| IBIS file imx8qm_29x29_rev1_27_15charsmax.ibs
[IBIS Ver]   6.0
[Comment Char]   |_char
[File Name]   imx8qm_29x29_rev1_27_15charsmax.ibs
[File Rev]   1.27
[Date]   Mon Mar 15 02:13:26 2021
[Source]   NXP Viper 2020.06.15
[Notes]
[Disclaimer] IMPORTANT NOTICE
  This information is provided on an AS IS basis and without warranty.
  IN NO EVENT SHALL NXP BE LIABLE FOR INCIDENTAL OR CONSEQUENTIAL
  DAMAGES ARISING FROM USE OF THIS INFORMATION. THIS DISCLAIMER OF
  WARRANTY EXTENDS TO THE USER OF THE INFORMATION, AND TO THEIR CUSTOMERS
  OR USERS OF PRODUCTS  AND IS IN LIEU OF ALL WARRANTIES WHETHER EXPRESS,
  IMPLIED, OR STATUTORY, INCLUDING IMPLIED WARRANTIES OF MERCHANTABILITY
  OR FITNESS FOR PARTICULAR PURPOSE.
  NXP does not represent or warrant that the information furnished
  hereunder is free of infringement of any third party patents,
  copyrights, trade secrets, or other intellectual property rights.
  NXP does not represent or warrant that the information is free of
  defect, or that it meets any particular standard, requirements or need
  of the user of the infomation or their customers.
  NXP reserves the right to change the information in this file
  without notice.
   http://www.nxp.com
[Copyright]   (C) Copyright NXP 2004 - 2021, All Rights Reserved.
|   29x29
[Component]   29x29
[Manufacturer]   NXP
[Package]
| variable   typ   min   max
R_pkg   0.50181   0.071251   0.87203
L_pkg   3.032e-09   8.667e-10   5.190e-09
C_pkg   1.442e-12   7.770e-13   2.498e-12
[Pin] signal_name   model_name   R_pin   L_pin   C_pin
A3   VSS_MAIN   GND   NA   NA   NA
A5   USDHC1_RESET_B   BDPROGSCARUDQP_SDMMC_STD_3V3SF_FC_INNER  0.71494   4.208e-09 1.803e-12
A7   USDHC2_VSELECT   BDPROGSCARUDQP_SDMMC_STD_3V3SF_FC_OUTER  0.67873   4.010e-09 1.761e-12
A9   ENET0_MDC   BDPROGSCARUDQP_SDMMC_STD_3V3SF_FC_OUTER  0.67049   4.031e-09 1.735e-12
A11   ENET1_REFCLK_125M_25M   BDPROGSCARUDQP_SDMMC_STD_3V3SF_FC_OUTER  0.64637   3.820e-09 1.719e-12
A13   ENET1_MDC   BDPROGSCARUDQP_SDMMC_STD_3V3SF_FC_OUTER  0.66667   3.947e-09 1.724e-12
A15   PCIE_CTRL0_WAKE_B   BDPROGSCARUDQP_SDMMC_STD_3V3SF_FC_OUTER  0.65437   3.912e-09 1.725e-12
A17   PCIE_CTRL0_CLKREQ_B   BDPROGSCARUDQP_SDMMC_STD_3V3SF_FC_INNER  0.68404   4.044e-09 1.697e-12
A19   PCIE_SATA0_RX0_P   ABI_SERDES   0.65685   4.000e-09 1.482e-12
A21   PCIE1_RX0_P   ABI_SERDES   0.61374   3.771e-09 1.410e-12
A23   VSS_MAIN   GND   NA   NA   NA
A25   PCIE_CTRL1_CLKREQ_B   BDPROGSCARUDQP_SDMMC_STD_3V3SF_FC_OUTER  0.85097   5.022e-09 2.136e-12
A27   PCIE_CTRL1_WAKE_B   BDPROGSCARUDQP_SDMMC_STD_3V3SF_FC_INNER  0.87203   5.190e-09 2.111e-12
A29   PCIE0_RX0_P   ABI_SERDES   0.60799   3.796e-09 1.403e-12
A31   VSS_MAIN   GND   NA   NA   NA
A33   USB_SS3_TX_P   USB3_CDN   0.57069   3.681e-09 1.574e-12
A35   USB_OTG2_VBUS   NC   0.74136   4.399e-09 1.861e-12
A37   USB_OTG1_ID   NC   0.82585   4.889e-09 1.965e-12
A39   USB_OTG1_VBUS   hs_vbus_input   0.79385   4.631e-09 1.953e-12
A41   ENET0_RGMII_TXC   BDPROGSCARUDQP_SDMMC_STD_3V3SF_FC_INNER  0.63855   3.785e-09 1.694e-12
A43   ENET0_RGMII_TXD0   BDPROGSCARUDQP_SDMMC_STD_3V3SF_FC_INNER  0.63821   3.801e-09 1.640e-12
A45   ENET0_RGMII_TXD2   BDPROGSCARUDQP_SDMMC_STD_3V3SF_FC_INNER  0.68513   3.981e-09 1.746e-12
A47   ENET0_RGMII_RXD0   BDPROGSCARUDQP_SDMMC_STD_3V3SF_FC_INNER  0.70942   4.117e-09 1.762e-12
A49   ENET1_RGMII_TXD0   RGMII_TX   0.70216   4.118e-09 1.784e-12
A51   VSS_MAIN   GND   NA   NA   NA
B4   USDHC1_VSELECT   BDPROGSCARUDQP_SDMMC_STD_3V3SF_FC_OUTER  0.72105   4.248e-09 1.878e-12
B6   VSS_MAIN   GND   NA   NA   NA
B8   USDHC2_CD_B   BDPROGSCARUDQP_SDMMC_STD_3V3SF_FC_OUTER  0.65725   3.867e-09 1.789e-12
B10   ENET0_REFCLK_125M_25M   BDPROGSCARUDQP_SDMMC_STD_3V3SF_FC_INNER  0.62462   3.773e-09 1.701e-12
B12   VSS_MAIN   GND   NA   NA   NA
B14   VSS_MAIN   GND   NA   NA   NA
B16   PCIE_SATA0_TX0_P   ABI_SERDES   0.66405   4.087e-09 1.502e-12
B18   VSS_MAIN   GND   NA   NA   NA
B20   PCIE_SATA0_RX0_N   ABI_SERDES   0.65179   3.969e-09 1.493e-12
B22   PCIE1_RX0_N   ABI_SERDES   0.60933   3.642e-09 1.423e-12
B24   PCIE1_TX0_P   ABI_SERDES   0.54832   3.450e-09 1.344e-12
B26   PCIE0_TX0_P   ABI_SERDES   0.53719   3.375e-09 1.333e-12
B28   VSS_MAIN   GND   NA   NA   NA
B30   PCIE0_RX0_N   ABI_SERDES   0.60644   3.657e-09 1.420e-12
B32   USB_SS3_TX_N   USB3_CDN   0.56535   3.654e-09 1.559e-12
B34   USB_SS3_RX_N   USB3_CDN   0.57636   3.751e-09 1.628e-12
B36   VSS_MAIN   GND   NA   NA   NA
B38   USB_OTG2_DP   USB2_CDN   0.66542   4.197e-09 1.802e-12
B40   USB_OTG1_DP   USB2_NXP   0.68855   4.331e-09 1.847e-12
B42   ENET0_RGMII_TXD1   BDPROGSCARUDQP_SDMMC_STD_3V3SF_FC_OUTER  0.58126   3.465e-09 1.663e-12
B44   ENET0_RGMII_RXC   BDPROGSCARUDQP_SDMMC_STD_3V3SF_FC_INNER  0.59473   3.532e-09 1.657e-12
B46   VSS_MAIN   GND   NA   NA   NA
B48   ENET1_RGMII_TX_CTL   RGMII_TX   0.67806   3.966e-09 1.806e-12
B50   ENET1_RGMII_RXC   RGMII_RX   0.6658   3.913e-09 1.811e-12
C1   VSS_MAIN   GND   NA   NA   NA
C3   FLEXCAN2_RX   BDPROGSCARUDQP_SDMMC_STD_3V3SF_FC_INNER  0.73333   4.310e-09 1.872e-12
C5   FLEXCAN0_RX   BDPROGSCARUDQP_SDMMC_STD_3V3SF_FC_INNER  0.6572   3.880e-09 1.799e-12
C7   USDHC2_RESET_B   BDPROGSCARUDQP_SDMMC_STD_3V3SF_FC_INNER  0.64223   3.776e-09 1.718e-12
C9   VSS_MAIN   GND   NA   NA   NA
C11   VSS_MAIN   GND   NA   NA   NA
C13   ENET1_MDIO   BDPROGSCARUDQP_SDMMC_STD_3V3SF_FC_INNER  0.63159   3.805e-09 1.707e-12
C15   VSS_MAIN   GND   NA   NA   NA
C17   PCIE_SATA0_TX0_N   ABI_SERDES   0.66021   3.964e-09 1.538e-12
C19   VSS_MAIN   GND   NA   NA   NA
C21   VSS_MAIN   GND   NA   NA   NA
C23   VSS_MAIN   GND   NA   NA   NA
C25   PCIE1_TX0_N   ABI_SERDES   0.54592   3.335e-09 1.359e-12
C27   PCIE0_TX0_N   ABI_SERDES   0.53539   3.267e-09 1.337e-12
C29   VSS_MAIN   GND   NA   NA   NA
C31   VSS_MAIN   GND   NA   NA   NA
C33   VSS_MAIN   GND   NA   NA   NA
C35   USB_SS3_RX_P   USB3_CDN   0.578   3.655e-09 1.644e-12
C37   USB_OTG2_DN   USB2_CDN   0.65338   4.100e-09 1.813e-12
C39   USB_OTG1_DN   USB2_NXP   0.68253   4.301e-09 1.869e-12
C41   VSS_MAIN   GND   NA   NA   NA
C43   VSS_MAIN   GND   NA   NA   NA
C45   ENET0_RGMII_RXD2   BDPROGSCARUDQP_SDMMC_STD_3V3SF_FC_INNER  0.56865   3.382e-09 1.610e-12
C47   ENET1_RGMII_TXD1   RGMII_TX   0.58297   3.447e-09 1.661e-12
C49   VSS_MAIN   GND   NA   NA   NA
C51   ENET1_RGMII_RXD1   RGMII_RX   0.69982   4.106e-09 1.867e-12
C53   VSS_MAIN   GND   NA   NA   NA
D2   MLB_CLK   BDPROGSCARUDQP_SDMMC_STD_3V3SF_FC_INNER  0.71101   4.209e-09 1.875e-12
D6   VSS_MAIN   GND   NA   NA   NA
D8   USDHC2_WP   BDPROGSCARUDQP_SDMMC_STD_3V3SF_FC_INNER  0.62513   3.651e-09 1.684e-12
D10   ENET0_MDIO   BDPROGSCARUDQP_SDMMC_STD_3V3SF_FC_INNER  0.56625   3.378e-09 1.592e-12
D12   QSPI1A_DATA0   BDPROGSCARUDQP_SDMMC_STD_3V3SF_FC_OUTER  0.56144   3.424e-09 1.570e-12
D14   QSPI1A_DATA1   BDPROGSCARUDQP_SDMMC_STD_3V3SF_FC_INNER  0.53085   3.195e-09 1.560e-12
D16   VSS_MAIN   GND   NA   NA   NA
D18   VSS_MAIN   GND   NA   NA   NA
D20   PCIE_CTRL0_PERST_B   BDPROGSCARUDQP_SDMMC_STD_3V3SF_FC_INNER  0.51533   3.133e-09 1.473e-12
D22   PCIE_REXT   NC   0.50872   3.207e-09 1.487e-12
D24   VSS_MAIN   GND   NA   NA   NA
D26   VSS_MAIN   GND   NA   NA   NA
D28   VSS_MAIN   GND   NA   NA   NA
D30   MLB_SIG_P   mlb_data   0.47295   2.889e-09 1.375e-12
D32   MLB_CLK_P   mlb_clk   0.47306   2.904e-09 1.407e-12
D34   VSS_MAIN   GND   NA   NA   NA
D36   VSS_MAIN   GND   NA   NA   NA
D38   VSS_MAIN   GND   NA   NA   NA
D40   VSS_MAIN   GND   NA   NA   NA
D42   ENET0_RGMII_TXD3   BDPROGSCARUDQP_SDMMC_STD_3V3SF_FC_OUTER  0.54802   3.277e-09 1.536e-12
D44   ENET0_RGMII_RXD1   BDPROGSCARUDQP_SDMMC_STD_3V3SF_FC_OUTER  0.54964   3.286e-09 1.569e-12
D46   ENET1_RGMII_TXC   RGMII_TX   0.56118   3.341e-09 1.609e-12
D48   ENET1_RGMII_TXD3   RGMII_TX   0.5816   3.434e-09 1.601e-12
D52   ENET1_RGMII_RXD2   RGMII_RX   0.67008   3.934e-09 1.799e-12
E1   MLB_SIG   BDPROGSCARUDQP_SDMMC_STD_3V3SF_FC_INNER  0.70584   4.172e-09 1.785e-12
E3   MLB_DATA   BDPROGSCARUDQP_SDMMC_STD_3V3SF_FC_OUTER  0.63145   3.764e-09 1.730e-12
E5   FLEXCAN1_RX   BDPROGSCARUDQP_SDMMC_STD_3V3SF_FC_INNER  0.60931   3.644e-09 1.672e-12
E7   FLEXCAN2_TX   BDPROGSCARUDQP_SDMMC_STD_3V3SF_FC_OUTER  0.54072   3.256e-09 1.551e-12
E9   VSS_MAIN   GND   NA   NA   NA
E11   QSPI1A_DATA3   BDPROGSCARUDQP_SDMMC_STD_3V3SF_FC_INNER  0.55954   3.390e-09 1.553e-12
E13   QSPI1A_DATA2   BDPROGSCARUDQP_SDMMC_STD_3V3SF_FC_OUTER  0.4728   2.874e-09 1.442e-12
E15   QSPI0A_SS0_B   BDPROGSCARUDQP_SDMMC_STD_3V3SF_FC_OUTER  0.51682   3.144e-09 1.446e-12
E17   QSPI0A_SCLK   BDPROGSCARUDQP_SDMMC_STD_3V3SF_FC_OUTER  0.44693   2.747e-09 1.424e-12
E19   VSS_MAIN   GND   NA   NA   NA
E21   VSS_MAIN   GND   NA   NA   NA
E23   PCIE_REF_QR   NC   0.44778   2.848e-09 1.371e-12
E25   PCIE_SATA_REFCLK100M_N   NC   0.45847   2.806e-09 1.335e-12
E27   USB_SS3_REXT   NC   0.43403   2.914e-09 1.329e-12
E29   USB_OTG2_REXT   NC   0.3739   2.509e-09 1.226e-12
E31   MLB_SIG_N   mlb_data   0.47898   2.890e-09 1.386e-12
E33   MLB_CLK_N   mlb_clk   0.48026   2.897e-09 1.367e-12
E35   MLB_DATA_N   mlb_data   0.50267   3.023e-09 1.406e-12
E37   USDHC1_DATA0   BDPROGSCARUDQP_SDMMC_STD_3V3SF_FC_OUTER  0.45646   2.769e-09 1.352e-12
E39   USDHC1_DATA2   BDPROGSCARUDQP_SDMMC_STD_3V3SF_FC_OUTER  0.50466   3.021e-09 1.399e-12
E41   ENET0_RGMII_TX_CTL   BDPROGSCARUDQP_SDMMC_STD_3V3SF_FC_OUTER  0.57458   3.399e-09 1.597e-12
E43   ENET0_RGMII_RX_CTL   BDPROGSCARUDQP_SDMMC_STD_3V3SF_FC_OUTER  0.52405   3.152e-09 1.459e-12
E45   ENET0_RGMII_RXD3   BDPROGSCARUDQP_SDMMC_STD_3V3SF_FC_OUTER  0.51175   3.076e-09 1.491e-12
E47   VSS_MAIN   GND   NA   NA   NA
E49   ENET1_RGMII_RX_CTL   RGMII_RX   0.60279   3.566e-09 1.646e-12
E51   ENET1_RGMII_RXD0   RGMII_RX   0.65133   3.797e-09 1.745e-12
E53   ENET1_RGMII_RXD3   RGMII_RX   0.68907   3.974e-09 1.824e-12
F2   VSS_MAIN   GND   NA   NA   NA
F4   VSS_MAIN   GND   NA   NA   NA
F8   USB_SS3_TC2   BDPROGSCUDQP_EXT_FC_INNER   0.52001   3.184e-09 1.481e-12
F10   QSPI1A_SCLK   BDPROGSCARUDQP_SDMMC_STD_3V3SF_FC_INNER  0.55245   3.337e-09 1.549e-12
F12   VSS_MAIN   GND   NA   NA   NA
F14   QSPI0A_DATA1   BDPROGSCARUDQP_SDMMC_STD_3V3SF_FC_OUTER  0.45208   2.741e-09 1.409e-12
F16   QSPI0A_SS1_B   BDPROGSCARUDQP_SDMMC_STD_3V3SF_FC_INNER  0.48133   2.964e-09 1.408e-12
F18   QSPI0B_SCLK   BDPROGSCARUDQP_SDMMC_STD_3V3SF_FC_INNER  0.39244   2.436e-09 1.330e-12
F20   QSPI0B_DATA3   BDPROGSCARUDQP_SDMMC_STD_3V3SF_FC_INNER  0.4028   2.469e-09 1.293e-12
F22   QSPI0B_SS0_B   BDPROGSCARUDQP_SDMMC_STD_3V3SF_FC_INNER  0.39427   2.450e-09 1.281e-12
F24   VSS_MAIN   GND   NA   NA   NA
F26   PCIE_SATA_REFCLK100M_P   NC   0.45666   2.807e-09 1.394e-12
F28   USB_HSIC0_STROBE   hsic   0.39203   2.462e-09 1.309e-12
F30   USB_OTG2_ID   NC   0.34712   2.212e-09 1.234e-12
F32   VSS_MAIN   GND   NA   NA   NA
F34   MLB_DATA_P   mlb_data   0.49658   3.005e-09 1.415e-12
F36   VSS_MAIN   GND   NA   NA   NA
F38   USDHC1_DATA1   BDPROGSCARUDQP_SDMMC_STD_3V3SF_FC_INNER  0.46305   2.802e-09 1.318e-12
F40   USDHC1_DATA3   BDPROGSCARUDQP_SDMMC_STD_3V3SF_FC_INNER  0.50226   3.028e-09 1.440e-12
F42   USDHC1_DATA6   BDPROGSCARUDQP_SDMMC_STD_3V3SF_FC_OUTER  0.47942   2.912e-09 1.417e-12
F44   VSS_MAIN   GND   NA   NA   NA
F46   USDHC2_CLK   BDPROGSCARUDQP_SDMMC_STD_3V3SF_FC_INNER  0.67177   4.003e-09 1.796e-12
F50   VSS_MAIN   GND   NA   NA   NA
F52   VSS_MAIN   GND   NA   NA   NA
G1   DDR_CH1_DQ05   PDDRIO_PAD_DATA   0.66326   3.933e-09 1.688e-12
G3   DDR_CH1_DQ06   PDDRIO_PAD_DATA   0.63448   3.859e-09 1.718e-12
G5   VSS_MAIN   GND   NA   NA   NA
G7   FLEXCAN1_TX   BDPROGSCARUDQP_SDMMC_STD_3V3SF_FC_OUTER  0.54812   3.301e-09 1.588e-12
G9   VSS_MAIN   GND   NA   NA   NA
G11   QSPI1A_SS1_B   BDPROGSCARUDQP_SDMMC_STD_3V3SF_FC_OUTER  0.48621   2.959e-09 1.523e-12
G13   QSPI0A_DATA0   BDPROGSCARUDQP_SDMMC_STD_3V3SF_FC_INNER  0.46056   2.802e-09 1.455e-12
G15   VSS_MAIN   GND   NA   NA   NA
G17   QSPI0A_DQS   BDPROGSCARUDQP_SDMMC_STD_3V3SF_FC_INNER  0.37077   2.353e-09 1.286e-12
G19   QSPI0B_DATA2   BDPROGSCARUDQP_SDMMC_STD_3V3SF_FC_OUTER  0.3765   2.329e-09 1.271e-12
G21   VSS_MAIN   GND   NA   NA   NA
G23   VSS_MAIN   GND   NA   NA   NA
G25   PCIE_CTRL1_PERST_B   BDPROGSCARUDQP_SDMMC_STD_3V3SF_FC_OUTER  0.33043   2.156e-09 1.186e-12
G27   VSS_MAIN   GND   NA   NA   NA
G29   EMMC0_DATA0   BDPROGSCARUDQP_SDMMC_STD_3V3SF_FC_INNER  0.412   2.597e-09 1.278e-12
G31   EMMC0_DATA2   BDPROGSCARUDQP_SDMMC_STD_3V3SF_FC_INNER  0.37909   2.358e-09 1.243e-12
G33   VSS_MAIN   GND   NA   NA   NA
G35   EMMC0_DATA7   BDPROGSCARUDQP_SDMMC_STD_3V3SF_FC_OUTER  0.35183   2.211e-09 1.183e-12
G37   EMMC0_STROBE   BDPROGSCARUDQP_SDMMC_STD_3V3SF_FC_INNER  0.37074   2.314e-09 1.244e-12
G39   VSS_MAIN   GND   NA   NA   NA
G41   USDHC1_CMD   BDPROGSCARUDQP_SDMMC_STD_3V3SF_FC_INNER  0.49738   2.969e-09 1.475e-12
G43   USDHC1_DATA5   BDPROGSCARUDQP_SDMMC_STD_3V3SF_FC_INNER  0.51832   3.079e-09 1.500e-12
G45   USDHC2_DATA1   BDPROGSCARUDQP_SDMMC_STD_3V3SF_FC_OUTER  0.5606   3.400e-09 1.610e-12
G47   ENET1_RGMII_TXD2   RGMII_TX   0.55697   3.297e-09 1.553e-12
G49   VSS_MAIN   GND   NA   NA   NA
G51   DDR_CH0_DQ06   PDDRIO_PAD_DATA   0.63199   3.750e-09 1.739e-12
G53   DDR_CH0_DQ05   PDDRIO_PAD_DATA   0.66027   3.881e-09 1.779e-12
H2   DDR_CH1_DM0   PDDRIO_PAD_DATA   0.62675   3.725e-09 1.662e-12
H4   DDR_CH1_DQ04   PDDRIO_PAD_DATA   0.56957   3.379e-09 1.592e-12
H6   FLEXCAN0_TX   BDPROGSCARUDQP_SDMMC_STD_3V3SF_FC_OUTER  0.53476   3.306e-09 1.585e-12
H10   USB_SS3_TC3   BDPROGSCUDQP_EXT_FC_OUTER   0.43538   2.704e-09 1.347e-12
H12   QSPI1A_DQS   BDPROGSCARUDQP_SDMMC_STD_3V3SF_FC_OUTER  0.43856   2.706e-09 1.408e-12
H14   QSPI0A_DATA2   BDPROGSCARUDQP_SDMMC_STD_3V3SF_FC_INNER  0.42256   2.614e-09 1.399e-12
H16   QSPI0A_DATA3   BDPROGSCARUDQP_SDMMC_STD_3V3SF_FC_OUTER  0.40728   2.516e-09 1.306e-12
H18   QSPI0B_DATA0   BDPROGSCARUDQP_SDMMC_STD_3V3SF_FC_OUTER  0.34663   2.215e-09 1.213e-12
H20   QSPI0B_DATA1   BDPROGSCARUDQP_SDMMC_STD_3V3SF_FC_INNER  0.31327   1.955e-09 1.168e-12
H22   QSPI0B_DQS   BDPROGSCARUDQP_SDMMC_STD_3V3SF_FC_OUTER  0.306   1.964e-09 1.132e-12
H24   QSPI0B_SS1_B   BDPROGSCARUDQP_SDMMC_STD_3V3SF_FC_OUTER  0.34933   2.209e-09 1.161e-12
H26   USB_HSIC0_DATA   hsic   0.29076   1.955e-09 1.108e-12
H28   EMMC0_CLK   BDPROGSCARUDQP_SDMMC_STD_3V3SF_FC_INNER  0.40001   2.468e-09 1.271e-12
H30   EMMC0_DATA1   BDPROGSCARUDQP_SDMMC_STD_3V3SF_FC_OUTER  0.35924   2.228e-09 1.208e-12
H32   EMMC0_DATA3   BDPROGSCARUDQP_SDMMC_STD_3V3SF_FC_OUTER  0.30585   1.968e-09 1.176e-12
H34   EMMC0_DATA5   BDPROGSCARUDQP_SDMMC_STD_3V3SF_FC_OUTER  0.33315   2.092e-09 1.130e-12
H36   EMMC0_DATA6   BDPROGSCARUDQP_SDMMC_STD_3V3SF_FC_INNER  0.35261   2.188e-09 1.178e-12
H38   EMMC0_RESET_B   BDPROGSCARUDQP_SDMMC_STD_3V3SF_FC_OUTER  0.38186   2.351e-09 1.248e-12
H40   USDHC1_DATA4   BDPROGSCARUDQP_SDMMC_STD_3V3SF_FC_OUTER  0.4384   2.664e-09 1.395e-12
H42   USDHC1_DATA7   BDPROGSCARUDQP_SDMMC_STD_3V3SF_FC_INNER  0.44709   2.716e-09 1.362e-12
H44   USDHC2_CMD   BDPROGSCARUDQP_SDMMC_STD_3V3SF_FC_OUTER  0.54162   3.262e-09 1.572e-12
H48   USDHC2_DATA0   BDPROGSCARUDQP_SDMMC_STD_3V3SF_FC_INNER  0.62353   3.680e-09 1.694e-12
H50   DDR_CH0_DQ04   PDDRIO_PAD_DATA   0.56734   3.363e-09 1.592e-12
H52   DDR_CH0_DM0   PDDRIO_PAD_DATA   0.62698   3.731e-09 1.687e-12
J1   VSS_MAIN   GND   NA   NA   NA
J3   VSS_MAIN   GND   NA   NA   NA
J5   VSS_MAIN   GND   NA   NA   NA
J7   VSS_MAIN   GND   NA   NA   NA
J9   USB_SS3_TC0   BDPROGSCUDQP_EXT_FC_INNER   0.42059   2.620e-09 1.335e-12
J11   QSPI1A_SS0_B   BDPROGSCARUDQP_SDMMC_STD_3V3SF_FC_INNER  0.49996   3.013e-09 1.556e-12
J13   VSS_MAIN   GND   NA   NA   NA
J15   VSS_MAIN   GND   NA   NA   NA
J17   VSS_MAIN   GND   NA   NA   NA
J19   VSS_MAIN   GND   NA   NA   NA
J21   VSS_MAIN   GND   NA   NA   NA
J23   VSS_MAIN   GND   NA   NA   NA
J25   VSS_MAIN   GND   NA   NA   NA
J27   EMMC0_CMD   BDPROGSCARUDQP_SDMMC_STD_3V3SF_FC_OUTER  0.37925   2.371e-09 1.227e-12
J29   VSS_MAIN   GND   NA   NA   NA
J31   VSS_MAIN   GND   NA   NA   NA
J33   EMMC0_DATA4   BDPROGSCARUDQP_SDMMC_STD_3V3SF_FC_INNER  0.31324   1.999e-09 1.165e-12
J35   VSS_MAIN   GND   NA   NA   NA
J37   VSS_MAIN   GND   NA   NA   NA
J39   USDHC1_CLK   BDPROGSCARUDQP_SDMMC_STD_3V3SF_FC_OUTER  0.38556   2.407e-09 1.236e-12
J41   VSS_MAIN   GND   NA   NA   NA
J43   USDHC1_STROBE   BDPROGSCARUDQP_SDMMC_STD_3V3SF_FC_OUTER  0.49046   2.949e-09 1.423e-12
J45   USDHC2_DATA3   BDPROGSCARUDQP_SDMMC_STD_3V3SF_FC_OUTER  0.52798   3.184e-09 1.404e-12
J47   VSS_MAIN   GND   NA   NA   NA
J49   VSS_MAIN   GND   NA   NA   NA
J51   VSS_MAIN   GND   NA   NA   NA
J53   VSS_MAIN   GND   NA   NA   NA
K2   DDR_CH1_DQS0_P   PDQS_PAD   0.72024   4.233e-09 1.841e-12
K4   DDR_CH1_DQ09   PDDRIO_PAD_DATA   0.54194   3.298e-09 1.528e-12
K6   DDR_CH1_DQ03   PDDRIO_PAD_DATA   0.48681   2.954e-09 1.443e-12
K8   VSS_MAIN   GND   NA   NA   NA
K12   VSS_MAIN   GND   NA   NA   NA
K14   VSS_MAIN   GND   NA   NA   NA
K16   VSS_MAIN   GND   NA   NA   NA
K18   VSS_MAIN   GND   NA   NA   NA
K20   VSS_MAIN   GND   NA   NA   NA
K22   VSS_MAIN   GND   NA   NA   NA
K24   VSS_MAIN   GND   NA   NA   NA
K26   VSS_MAIN   GND   NA   NA   NA
K28   VSS_MAIN   GND   NA   NA   NA
K30   VSS_MAIN   GND   NA   NA   NA
K32   VSS_MAIN   GND   NA   NA   NA
K34   VSS_MAIN   GND   NA   NA   NA
K36   VSS_MAIN   GND   NA   NA   NA
K38   VSS_MAIN   GND   NA   NA   NA
K40   VSS_MAIN   GND   NA   NA   NA
K42   VSS_MAIN   GND   NA   NA   NA
K46   VSS_MAIN   GND   NA   NA   NA
K48   DDR_CH0_DQ03   PDDRIO_PAD_DATA   0.48777   2.944e-09 1.414e-12
K50   DDR_CH0_DQ09   PDDRIO_PAD_DATA   0.54335   3.312e-09 1.488e-12
K52   DDR_CH0_DQS0_P   PDQS_PAD   0.72197   4.255e-09 1.844e-12
L1   DDR_CH1_DQS0_N   PDQS_PAD   0.72434   4.328e-09 1.757e-12
L3   DDR_CH1_DQ11   PDDRIO_PAD_DATA   0.59817   3.687e-09 1.610e-12
L5   DDR_CH1_DQ08   PDDRIO_PAD_DATA   0.48028   2.943e-09 1.425e-12
L7   DDR_CH1_DQ02   PDDRIO_PAD_DATA   0.45079   2.788e-09 1.323e-12
L9   USB_SS3_TC1   BDPROGSCUDQP_EXT_FC_OUTER   0.39437   2.514e-09 1.317e-12
L11   VSS_MAIN   GND   NA   NA   NA
L13   VSS_MAIN   GND   NA   NA   NA
L15   VSS_MAIN   GND   NA   NA   NA
L17   VSS_MAIN   GND   NA   NA   NA
L19   VSS_MAIN   GND   NA   NA   NA
L21   VSS_MAIN   GND   NA   NA   NA
L23   VSS_MAIN   GND   NA   NA   NA
L25   VSS_MAIN   GND   NA   NA   NA
L27   VSS_MAIN   GND   NA   NA   NA
L29   VSS_MAIN   GND   NA   NA   NA
L31   VSS_MAIN   GND   NA   NA   NA
L33   VSS_MAIN   GND   NA   NA   NA
L35   VSS_MAIN   GND   NA   NA   NA
L37   VSS_MAIN   GND   NA   NA   NA
L39   VSS_MAIN   GND   NA   NA   NA
L41   VSS_MAIN   GND   NA   NA   NA
L43   VSS_MAIN   GND   NA   NA   NA
L45   USDHC2_DATA2   BDPROGSCARUDQP_SDMMC_STD_3V3SF_FC_INNER  0.45871   2.725e-09 1.411e-12
L47   DDR_CH0_DQ02   PDDRIO_PAD_DATA   0.45083   2.841e-09 1.355e-12
L49   DDR_CH0_DQ08   PDDRIO_PAD_DATA   0.48155   2.926e-09 1.418e-12
L51   DDR_CH0_DQ11   PDDRIO_PAD_DATA   0.59934   3.648e-09 1.622e-12
L53   DDR_CH0_DQS0_N   PDQS_PAD   0.7235   4.319e-09 1.771e-12
M2   VSS_MAIN   GND   NA   NA   NA
M4   VSS_MAIN   GND   NA   NA   NA
M6   VSS_MAIN   GND   NA   NA   NA
M8   VSS_MAIN   GND   NA   NA   NA
M10   VSS_MAIN   GND   NA   NA   NA
M14   VDD_MLB_DIG_1P8_3P3   POWER   NA   NA   NA
M16   VDD_USB_SS3_TC_3P3   POWER   NA   NA   NA
M18   VDD_QSPI1A_1P8_3P3   POWER   NA   NA   NA
M20   PCIE_SATA0_PHY_PLL_REF_RETURN   GND   0.078076  8.883e-10 2.121e-12
M22   VDD_PCIE1_PLL_1P8   POWER   NA   NA   NA
M24   VDD_PCIE_SATA0_1P0   POWER   NA   NA   NA
M26   VDD_PCIE0_1P0   POWER   NA   NA   NA
M28   PCIE0_PHY_PLL_REF_RETURN   GND   0.090376  9.966e-10 1.927e-12
M30   VDD_USB_SS3_LDO_1P0_CAP   POWER   NA   NA   NA
M32   VDD_USB_OTG1_1P0   POWER   NA   NA   NA
M34   VDD_USB_OTG2_3P3   POWER   NA   NA   NA
M36   VDD_USDHC1_1P8_3P3   POWER   NA   NA   NA
M38   VDD_USDHC2_1P8_3P3   POWER   NA   NA   NA
M40   VDD_ENET0_1P8_2P5_3P3   POWER   NA   NA   NA
M44   VSS_MAIN   GND   NA   NA   NA
M46   VSS_MAIN   GND   NA   NA   NA
M48   VSS_MAIN   GND   NA   NA   NA
M50   VSS_MAIN   GND   NA   NA   NA
M52   VSS_MAIN   GND   NA   NA   NA
N1   DDR_CH1_DQS1_P   PDQS_PAD   0.6386   3.872e-09 1.642e-12
N3   DDR_CH1_DQ10   PDDRIO_PAD_DATA   0.54172   3.267e-09 1.538e-12
N5   DDR_CH1_DQ13   PDDRIO_PAD_DATA   0.45905   2.855e-09 1.364e-12
N7   DDR_CH1_DM1   PDDRIO_PAD_DATA   0.3749   2.404e-09 1.248e-12
N9   DDR_CH1_DQ01   PDDRIO_PAD_DATA   0.31995   2.039e-09 1.116e-12
N11   DDR_CH1_DQ07   PDDRIO_PAD_DATA   0.23187   1.570e-09 9.871e-13
N13   VSS_MAIN   GND   NA   NA   NA
N15   VDD_FLEXCAN_1P8_3P3   POWER   NA   NA   NA
N17   VDD_ENET_MDIO_1P8_2P5_3P3   POWER   NA   NA   NA
N19   VDD_QSPI0_1P8_3P3   POWER   NA   NA   NA
N21   VDD_PCIE_SATA0_PLL_1P8   POWER   NA   NA   NA
N23   PCIE1_PHY_PLL_REF_RETURN   GND   0.072195  9.525e-10 1.343e-12
N25   VDD_PCIE1_1P0   POWER   NA   NA   NA
N27   VDD_PCIE0_PLL_1P8   POWER   NA   NA   NA
N29   VDD_PCIE_LDO_1P0_CAP   POWER   NA   NA   NA
N31   VDD_USB_OTG2_1P0   POWER   NA   NA   NA
N33   VDD_USB_OTG1_3P3   POWER   NA   NA   NA
N35   VDD_EMMC0_1P8_3P3   POWER   NA   NA   NA
N37   VDD_USDHC1_1P8_3P3   POWER   NA   NA   NA
N39   VDD_ENET0_1P8_2P5_3P3   POWER   NA   NA   NA
N41   VSS_MAIN   GND   NA   NA   NA
N43   DDR_CH0_DQ07   PDDRIO_PAD_DATA   0.22999   1.544e-09 9.890e-13
N45   DDR_CH0_DQ01   PDDRIO_PAD_DATA   0.32072   2.032e-09 1.120e-12
N47   DDR_CH0_DM1   PDDRIO_PAD_DATA   0.37407   2.370e-09 1.247e-12
N49   DDR_CH0_DQ13   PDDRIO_PAD_DATA   0.46598   2.903e-09 1.391e-12
N51   DDR_CH0_DQ10   PDDRIO_PAD_DATA   0.54312   3.246e-09 1.498e-12
N53   DDR_CH0_DQS1_P   PDQS_PAD   0.63588   3.825e-09 1.623e-12
P2   DDR_CH1_DQS1_N   PDQS_PAD   0.62973   3.778e-09 1.665e-12
P4   DDR_CH1_DQ14   PDDRIO_PAD_DATA   0.47322   2.923e-09 1.416e-12
P6   DDR_CH1_DQ15   PDDRIO_PAD_DATA   0.41122   2.633e-09 1.290e-12
P8   DDR_CH1_DQ12   PDDRIO_PAD_DATA   0.31879   2.070e-09 1.140e-12
P10   DDR_CH1_DQ00   PDDRIO_PAD_DATA   0.26612   1.777e-09 1.004e-12
P12   VSS_MAIN   GND   NA   NA   NA
P42   VSS_MAIN   GND   NA   NA   NA
P44   DDR_CH0_DQ00   PDDRIO_PAD_DATA   0.26606   1.803e-09 9.926e-13
P46   DDR_CH0_DQ12   PDDRIO_PAD_DATA   0.31564   1.974e-09 1.142e-12
P48   DDR_CH0_DQ15   PDDRIO_PAD_DATA   0.42142   2.670e-09 1.295e-12
P50   DDR_CH0_DQ14   PDDRIO_PAD_DATA   0.47632   2.946e-09 1.401e-12
P52   DDR_CH0_DQS1_N   PDQS_PAD   0.6299   3.763e-09 1.657e-12
R1   VSS_MAIN   GND   NA   NA   NA
R3   VSS_MAIN   GND   NA   NA   NA
R5   VSS_MAIN   GND   NA   NA   NA
R7   VSS_MAIN   GND   NA   NA   NA
R9   VSS_MAIN   GND   NA   NA   NA
R11   VSS_MAIN   GND   NA   NA   NA
R15   VSS_MAIN   GND   NA   NA   NA
R17   VSS_MAIN   GND   NA   NA   NA
R19   VSS_MAIN   GND   NA   NA   NA
R21   VSS_MAIN   GND   NA   NA   NA
R23   VSS_MAIN   GND   NA   NA   NA
R25   VSS_MAIN   GND   NA   NA   NA
R27   VSS_MAIN   GND   NA   NA   NA
R29   VSS_MAIN   GND   NA   NA   NA
R31   VSS_MAIN   GND   NA   NA   NA
R33   VSS_MAIN   GND   NA   NA   NA
R35   VSS_MAIN   GND   NA   NA   NA
R37   VSS_MAIN   GND   NA   NA   NA
R39   VSS_MAIN   GND   NA   NA   NA
R43   VSS_MAIN   GND   NA   NA   NA
R45   VSS_MAIN   GND   NA   NA   NA
R47   VSS_MAIN   GND   NA   NA   NA
R49   VSS_MAIN   GND   NA   NA   NA
R51   VSS_MAIN   GND   NA   NA   NA
R53   VSS_MAIN   GND   NA   NA   NA
T2   DDR_CH1_DCF09   PDDRIO_PAD_COMMAND   0.54813   3.276e-09 1.456e-12
T4   DDR_CH1_DCF10   PDDRIO_PAD_COMMAND   0.45838   2.772e-09 1.396e-12
T6   DDR_CH1_DCF08   PDDRIO_PAD_COMMAND   0.4138   2.542e-09 1.341e-12
T8   DDR_CH1_DCF13   PDDRIO_PAD_COMMAND   0.37803   2.393e-09 1.184e-12
T10   DDR_CH1_DTO1   PDDRIO_PAD_COMMAND   0.32279   2.073e-09 1.114e-12
T12   VSS_MAIN   GND   NA   NA   NA
T16   VSS_MAIN   GND   NA   NA   NA
T18   VDD_USDHC_VSELECT_1P8_3P3   POWER   NA   NA   NA
T20   VSS_MAIN   GND   NA   NA   NA
T22   VDD_PCIE_DIG_1P8_3P3   POWER   NA   NA   NA
T24   VSS_MAIN   GND   NA   NA   NA
T26   VDD_PCIE_IOB_1P8   POWER   NA   NA   NA
T28   VSS_MAIN   GND   NA   NA   NA
T30   VDD_MLB_1P8   POWER   NA   NA   NA
T32   VSS_MAIN   GND   NA   NA   NA
T34   VDD_MAIN   POWER   NA   NA   NA
T36   VSS_MAIN   GND   NA   NA   NA
T38   VDD_ENET1_1P8_2P5_3P3   POWER   NA   NA   NA
T42   VSS_MAIN   GND   NA   NA   NA
T44   DDR_CH0_DTO1   PDDRIO_PAD_COMMAND   0.32378   2.069e-09 1.115e-12
T46   DDR_CH0_DCF13   PDDRIO_PAD_COMMAND   0.37542   2.342e-09 1.191e-12
T48   DDR_CH0_DCF08   PDDRIO_PAD_COMMAND   0.41391   2.551e-09 1.300e-12
T50   DDR_CH0_DCF10   PDDRIO_PAD_COMMAND   0.45654   2.774e-09 1.396e-12
T52   DDR_CH0_DCF09   PDDRIO_PAD_COMMAND   0.54626   3.230e-09 1.570e-12
U1   DDR_CH1_DCF16   PDDRIO_PAD_COMMAND   0.54739   3.303e-09 1.529e-12
U3   DDR_CH1_DCF11   PDDRIO_PAD_COMMAND   0.5197   3.133e-09 1.489e-12
U5   DDR_CH1_DCF12   PDDRIO_PAD_COMMAND   0.42237   2.576e-09 1.387e-12
U7   DDR_CH1_DCF00   PDDRIO_PAD_COMMAND   0.35953   2.250e-09 1.250e-12
U9   DDR_CH1_DTO0   PDDRIO_PAD_COMMAND   0.24832   1.674e-09 9.811e-13
U11   DDR_CH1_VREF   NC   0.071251  8.720e-10 2.474e-12
U15   VDD_DDR_CH1_VDDQ   POWER   NA   NA   NA
U17   VSS_MAIN   GND   NA   NA   NA
U19   VDD_MAIN   POWER   NA   NA   NA
U21   VSS_MAIN   GND   NA   NA   NA
U23   VDD_MAIN   POWER   NA   NA   NA
U25   VDD_ANA1_1P8   POWER   NA   NA   NA
U27   VDD_PCIE_LDO_1P8   POWER   NA   NA   NA
U29   VDD_ANA0_1P8   POWER   NA   NA   NA
U31   VDD_ANA0_1P8   POWER   NA   NA   NA
U33   VSS_MAIN   GND   NA   NA   NA
U35   VDD_GPU1   POWER   NA   NA   NA
U37   VSS_MAIN   GND   NA   NA   NA
U39   VDD_DDR_CH0_VDDQ   POWER   NA   NA   NA
U43   DDR_CH0_VREF   NC   0.072272  8.667e-10 2.439e-12
U45   DDR_CH0_DTO0   PDDRIO_PAD_COMMAND   0.24706   1.642e-09 9.813e-13
U47   DDR_CH0_DCF00   PDDRIO_PAD_COMMAND   0.35996   2.249e-09 1.228e-12
U49   DDR_CH0_DCF12   PDDRIO_PAD_COMMAND   0.42158   2.584e-09 1.355e-12
U51   DDR_CH0_DCF11   PDDRIO_PAD_COMMAND   0.51885   3.098e-09 1.498e-12
U53   DDR_CH0_DCF16   PDDRIO_PAD_COMMAND   0.54668   3.217e-09 1.515e-12
V2   VSS_MAIN   GND   NA   NA   NA
V4   VSS_MAIN   GND   NA   NA   NA
V6   VSS_MAIN   GND   NA   NA   NA
V8   VSS_MAIN   GND   NA   NA   NA
V10   VSS_MAIN   GND   NA   NA   NA
V12   VSS_MAIN   GND   NA   NA   NA
V16   VDD_DDR_CH1_VDDQ   POWER   NA   NA   NA
V18   VSS_MAIN   GND   NA   NA   NA
V20   VDD_GPU0   POWER   NA   NA   NA
V22   VSS_MAIN   GND   NA   NA   NA
V24   VDD_MAIN   POWER   NA   NA   NA
V26   VDD_USB_HSIC0_1P2   POWER   NA   NA   NA
V28   VDD_USB_HSIC0_1P8   POWER   NA   NA   NA
V30   VSS_MAIN   GND   NA   NA   NA
V32   VDD_MAIN   POWER   NA   NA   NA
V34   VSS_MAIN   GND   NA   NA   NA
V36   VDD_GPU1   POWER   NA   NA   NA
V38   VDD_DDR_CH0_VDDQ   POWER   NA   NA   NA
V42   VSS_MAIN   GND   NA   NA   NA
V44   VSS_MAIN   GND   NA   NA   NA
V46   VSS_MAIN   GND   NA   NA   NA
V48   VSS_MAIN   GND   NA   NA   NA
V50   VSS_MAIN   GND   NA   NA   NA
V52   VSS_MAIN   GND   NA   NA   NA
W1   DDR_CH1_DCF14   PCKE_PAD   0.60482   3.621e-09 1.615e-12
W3   DDR_CH1_DCF07   PDDRIO_PAD_COMMAND   0.4918   3.003e-09 1.518e-12
W5   DDR_CH1_CK0_P   PCK_PAD   0.53958   3.259e-09 1.520e-12
W7   DDR_CH1_DCF01   PDDRIO_PAD_COMMAND   0.33952   2.117e-09 1.220e-12
W9   DDR_CH1_DCF06   PDDRIO_PAD_COMMAND   0.33867   2.188e-09 1.127e-12
W11   DDR_CH1_DCF04   PDDRIO_PAD_COMMAND   0.28644   1.870e-09 1.056e-12
W15   VDD_DDR_CH1_VDDQ   POWER   NA   NA   NA
W17   VDD_MEMC   POWER   NA   NA   NA
W19   VSS_MAIN   GND   NA   NA   NA
W21   VDD_GPU0   POWER   NA   NA   NA
W23   VSS_MAIN   GND   NA   NA   NA
W25   VDD_MAIN   POWER   NA   NA   NA
W27   VSS_MAIN   GND   NA   NA   NA
W29   VDD_MAIN   POWER   NA   NA   NA
W31   VSS_MAIN   GND   NA   NA   NA
W33   VDD_GPU1   POWER   NA   NA   NA
W35   VSS_MAIN   GND   NA   NA   NA
W37   VDD_MEMC   POWER   NA   NA   NA
W39   VDD_DDR_CH0_VDDQ   POWER   NA   NA   NA
W43   DDR_CH0_DCF04   PDDRIO_PAD_COMMAND   0.28234   1.820e-09 1.133e-12
W45   DDR_CH0_DCF06   PDDRIO_PAD_COMMAND   0.34021   2.038e-09 1.116e-12
W47   DDR_CH0_DCF01   PDDRIO_PAD_COMMAND   0.33863   2.129e-09 1.222e-12
W49   DDR_CH0_CK0_P   PCK_PAD   0.54112   3.246e-09 1.529e-12
W51   DDR_CH0_DCF07   PDDRIO_PAD_COMMAND   0.49015   2.964e-09 1.471e-12
W53   DDR_CH0_DCF14   PCKE_PAD   0.6024   3.590e-09 1.616e-12
Y2   DDR_CH1_DCF15   PCKE_PAD   0.67035   3.910e-09 1.766e-12
Y4   DDR_CH1_CK0_N   PCK_PAD   0.55141   3.334e-09 1.523e-12
Y6   DDR_CH1_DCF02   PDDRIO_PAD_COMMAND   0.40922   2.543e-09 1.283e-12
Y8   DDR_CH1_DCF03   PDDRIO_PAD_COMMAND   0.30587   1.925e-09 1.080e-12
Y10   DDR_CH1_DCF05   PDDRIO_PAD_COMMAND   0.28611   1.870e-09 1.075e-12
Y12   VSS_MAIN   GND   NA   NA   NA
Y16   VDD_DDR_CH1_VDDQ   POWER   NA   NA   NA
Y18   VDD_GPU0   POWER   NA   NA   NA
Y20   VSS_MAIN   GND   NA   NA   NA
Y22   VDD_GPU0   POWER   NA   NA   NA
Y24   VSS_MAIN   GND   NA   NA   NA
Y26   VDD_MAIN   POWER   NA   NA   NA
Y28   VSS_MAIN   GND   NA   NA   NA
Y30   VDD_MAIN   POWER   NA   NA   NA
Y32   VSS_MAIN   GND   NA   NA   NA
Y34   VDD_GPU1   POWER   NA   NA   NA
Y36   VSS_MAIN   GND   NA   NA   NA
Y38   VDD_DDR_CH0_VDDQ   POWER   NA   NA   NA
Y42   VSS_MAIN   GND   NA   NA   NA
Y44   DDR_CH0_DCF05   PDDRIO_PAD_COMMAND   0.28056   1.802e-09 1.116e-12
Y46   DDR_CH0_DCF03   PDDRIO_PAD_COMMAND   0.30517   1.875e-09 1.073e-12
Y48   DDR_CH0_DCF02   PDDRIO_PAD_COMMAND   0.41107   2.514e-09 1.285e-12
Y50   DDR_CH0_CK0_N   PCK_PAD   0.54805   3.264e-09 1.522e-12
Y52   DDR_CH0_DCF15   PCKE_PAD   0.67128   3.926e-09 1.746e-12
AA1   VSS_MAIN   GND   NA   NA   NA
AA3   VSS_MAIN   GND   NA   NA   NA
AA5   VSS_MAIN   GND   NA   NA   NA
AA7   VSS_MAIN   GND   NA   NA   NA
AA9   VSS_MAIN   GND   NA   NA   NA
AA11  VSS_MAIN   GND   NA   NA   NA
AA13  VSS_MAIN   GND   NA   NA   NA
AA15  VDD_DDR_CH1_VDDQ   POWER   NA   NA   NA
AA17  VSS_MAIN   GND   NA   NA   NA
AA19  VDD_GPU0   POWER   NA   NA   NA
AA21  VSS_MAIN   GND   NA   NA   NA
AA23  VDD_MAIN   POWER   NA   NA   NA
AA25  VSS_MAIN   GND   NA   NA   NA
AA27  VDD_MAIN   POWER   NA   NA   NA
AA29  VSS_MAIN   GND   NA   NA   NA
AA31  VDD_MAIN   POWER   NA   NA   NA
AA33  VSS_MAIN   GND   NA   NA   NA
AA35  VDD_GPU1   POWER   NA   NA   NA
AA37  VSS_MAIN   GND   NA   NA   NA
AA39  VDD_DDR_CH0_VDDQ   POWER   NA   NA   NA
AA41  VSS_MAIN   GND   NA   NA   NA
AA43  VSS_MAIN   GND   NA   NA   NA
AA45  VSS_MAIN   GND   NA   NA   NA
AA47  VSS_MAIN   GND   NA   NA   NA
AA49  VSS_MAIN   GND   NA   NA   NA
AA51  VSS_MAIN   GND   NA   NA   NA
AA53  VSS_MAIN   GND   NA   NA   NA
AB2   DDR_CH1_DCF31   PCKE_PAD   0.65896   3.981e-09 1.723e-12
AB4   DDR_CH1_CK1_N   PCK_PAD   0.47431   2.952e-09 1.376e-12
AB6   DDR_CH1_DCF18   PCKE_PAD   0.36824   2.324e-09 1.233e-12
AB8   DDR_CH1_DCF19   PDDRIO_PAD_COMMAND   0.33456   2.091e-09 1.171e-12
AB10  DDR_CH1_DCF24   PDDRIO_PAD_COMMAND   0.30072   2.002e-09 1.096e-12
AB12  VSS_MAIN   GND   NA   NA   NA
AB16  VDD_DDR_CH1_VDDQ_CKE   POWER   NA   NA   NA
AB18  VSS_MAIN   GND   NA   NA   NA
AB20  VDD_GPU0   POWER   NA   NA   NA
AB22  VSS_MAIN   GND   NA   NA   NA
AB24  VDD_MAIN   POWER   NA   NA   NA
AB26  VSS_MAIN   GND   NA   NA   NA
AB28  VDD_MAIN   POWER   NA   NA   NA
AB30  VSS_MAIN   GND   NA   NA   NA
AB32  VDD_GPU1   POWER   NA   NA   NA
AB34  VSS_MAIN   GND   NA   NA   NA
AB36  VDD_GPU1   POWER   NA   NA   NA
AB38  VDD_DDR_CH0_VDDQ_CKE   POWER   NA   NA   NA
AB42  VSS_MAIN   GND   NA   NA   NA
AB44  DDR_CH0_DCF24   PDDRIO_PAD_COMMAND   0.3045   1.920e-09 1.124e-12
AB46  DDR_CH0_DCF19   PDDRIO_PAD_COMMAND   0.33395   2.111e-09 1.149e-12
AB48  DDR_CH0_DCF18   PCKE_PAD   0.36795   2.328e-09 1.201e-12
AB50  DDR_CH0_CK1_N   PCK_PAD   0.47459   2.903e-09 1.378e-12
AB52  DDR_CH0_DCF31   PCKE_PAD   0.65989   3.986e-09 1.745e-12
AC1   DDR_CH1_DCF30   PCKE_PAD   0.50721   3.093e-09 1.409e-12
AC3   DDR_CH1_DCF22   PDDRIO_PAD_COMMAND   0.49781   3.005e-09 1.407e-12
AC5   DDR_CH1_CK1_P   PCK_PAD   0.46603   2.874e-09 1.378e-12
AC7   DDR_CH1_DCF17   PDDRIO_PAD_COMMAND   0.29578   1.900e-09 1.089e-12
AC9   DDR_CH1_DCF23   PDDRIO_PAD_COMMAND   0.23551   1.560e-09 9.407e-13
AC11  DDR_CH1_DCF20   PDDRIO_PAD_COMMAND   0.15882   1.232e-09 8.141e-13
AC13  VSS_MAIN   GND   NA   NA   NA
AC15  VDD_DDR_CH1_VDDQ_CKE   POWER   NA   NA   NA
AC17  VDD_MEMC   POWER   NA   NA   NA
AC19  VSS_MAIN   GND   NA   NA   NA
AC21  VDD_GPU0   POWER   NA   NA   NA
AC23  VSS_MAIN   GND   NA   NA   NA
AC25  VDD_MAIN   POWER   NA   NA   NA
AC27  VSS_MAIN   GND   NA   NA   NA
AC29  VDD_MAIN   POWER   NA   NA   NA
AC31  VSS_MAIN   GND   NA   NA   NA
AC33  VDD_GPU1   POWER   NA   NA   NA
AC35  VSS_MAIN   GND   NA   NA   NA
AC37  VDD_MEMC   POWER   NA   NA   NA
AC39  VDD_DDR_CH0_VDDQ_CKE   POWER   NA   NA   NA
AC41  VSS_MAIN   GND   NA   NA   NA
AC43  DDR_CH0_DCF20   PDDRIO_PAD_COMMAND   0.15541   1.210e-09 8.215e-13
AC45  DDR_CH0_DCF23   PDDRIO_PAD_COMMAND   0.23204   1.507e-09 9.442e-13
AC47  DDR_CH0_DCF17   PDDRIO_PAD_COMMAND   0.29645   1.925e-09 1.065e-12
AC49  DDR_CH0_CK1_P   PCK_PAD   0.4672   2.863e-09 1.378e-12
AC51  DDR_CH0_DCF22   PDDRIO_PAD_COMMAND   0.49607   2.964e-09 1.462e-12
AC53  DDR_CH0_DCF30   PCKE_PAD   0.50593   3.073e-09 1.406e-12
AD2   VSS_MAIN   GND   NA   NA   NA
AD4   VSS_MAIN   GND   NA   NA   NA
AD6   VSS_MAIN   GND   NA   NA   NA
AD8   VSS_MAIN   GND   NA   NA   NA
AD10  VSS_MAIN   GND   NA   NA   NA
AD12  VSS_MAIN   GND   NA   NA   NA
AD16  VDD_DDR_CH1_VDDQ_CKE   POWER   NA   NA   NA
AD18  VDD_GPU0   POWER   NA   NA   NA
AD20  VSS_MAIN   GND   NA   NA   NA
AD22  VDD_GPU0   POWER   NA   NA   NA
AD24  VSS_MAIN   GND   NA   NA   NA
AD26  VDD_MAIN   POWER   NA   NA   NA
AD28  VSS_MAIN   GND   NA   NA   NA
AD30  VDD_MAIN   POWER   NA   NA   NA
AD32  VSS_MAIN   GND   NA   NA   NA
AD34  VDD_GPU1   POWER   NA   NA   NA
AD36  VSS_MAIN   GND   NA   NA   NA
AD38  VDD_DDR_CH0_VDDQ_CKE   POWER   NA   NA   NA
AD42  VSS_MAIN   GND   NA   NA   NA
AD44  VSS_MAIN   GND   NA   NA   NA
AD46  VSS_MAIN   GND   NA   NA   NA
AD48  VSS_MAIN   GND   NA   NA   NA
AD50  VSS_MAIN   GND   NA   NA   NA
AD52  VSS_MAIN   GND   NA   NA   NA
AE1   DDR_CH1_DCF32   PDDRIO_PAD_COMMAND   0.56662   3.425e-09 1.517e-12
AE3   DDR_CH1_DCF27   PDDRIO_PAD_COMMAND   0.46973   2.832e-09 1.413e-12
AE5   DDR_CH1_DCF29   PDDRIO_PAD_COMMAND   0.39873   2.478e-09 1.266e-12
AE7   DDR_CH1_DCF26   PDDRIO_PAD_COMMAND   0.37771   2.348e-09 1.197e-12
AE9   DDR_CH1_DCF21   PDDRIO_PAD_COMMAND   0.2605   1.722e-09 1.079e-12
AE11  VDD_DDR_CH1_VDDA_PLL_1P8   POWER   NA   NA   NA
AE13  VSS_MAIN   GND   NA   NA   NA
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[Pin Mapping]   pulldown_ref   pullup_ref
A3   VSS_MAIN   NC
A5   VSS_MAIN   VDDUSDHCVSELECT
A7   VSS_MAIN   VDDUSDHCVSELECT
A9   VSS_MAIN   VDDENET_MDIO
A11   VSS_MAIN   VDDENET_MDIO
A13   VSS_MAIN   VDDENET_MDIO
A15   VSS_MAIN   VDDPCIE_DIG
A17   VSS_MAIN   VDDPCIE_DIG
A19   VSS_MAIN   VDD_SATA0_1P0
A21   VSS_MAIN   VDD_PCIE1_1P0
A23   VSS_MAIN   NC
A25   VSS_MAIN   VDDPCIE_DIG
A27   VSS_MAIN   VDDPCIE_DIG
A29   VSS_MAIN   VDD_PCIE0_1P0
A31   VSS_MAIN   NC
A33   VSS_MAIN   VDD_ANA0_1P8
A35   NC   NC
A37   NC   NC
A39   VSS_MAIN   NC
A41   VSS_MAIN   VDD_ENET0
A43   VSS_MAIN   VDD_ENET0
A45   VSS_MAIN   VDD_ENET0
A47   VSS_MAIN   VDD_ENET0
A49   VSS_MAIN   VDD_ENET1
A51   VSS_MAIN   NC
B4   VSS_MAIN   VDDUSDHCVSELECT
B6   VSS_MAIN   NC
B8   VSS_MAIN   VDDUSDHCVSELECT
B10   VSS_MAIN   VDDENET_MDIO
B12   VSS_MAIN   NC
B14   VSS_MAIN   NC
B16   VSS_MAIN   VDD_SATA0_1P0
B18   VSS_MAIN   NC
B20   VSS_MAIN   VDD_SATA0_1P0
B22   VSS_MAIN   VDD_PCIE1_1P0
B24   VSS_MAIN   VDD_PCIE1_1P0
B26   VSS_MAIN   VDD_PCIE0_1P0
B28   VSS_MAIN   NC
B30   VSS_MAIN   VDD_PCIE0_1P0
B32   VSS_MAIN   VDD_ANA0_1P8
B34   VSS_MAIN   VDD_ANA0_1P8
B36   VSS_MAIN   NC
B38   VSS_MAIN   VDDUSBOTG2_3P3
B40   VSS_MAIN   VDDUSBOTG1_3P3
B42   VSS_MAIN   VDD_ENET0
B44   VSS_MAIN   VDD_ENET0
B46   VSS_MAIN   NC
B48   VSS_MAIN   VDD_ENET1
B50   VSS_MAIN   VDD_ENET1
C1   VSS_MAIN   NC
C3   VSS_MAIN   VDDFLEXCAN
C5   VSS_MAIN   VDDFLEXCAN
C7   VSS_MAIN   VDDUSDHCVSELECT
C9   VSS_MAIN   NC
C11   VSS_MAIN   NC
C13   VSS_MAIN   VDDENET_MDIO
C15   VSS_MAIN   NC
C17   VSS_MAIN   VDD_SATA0_1P0
C19   VSS_MAIN   NC
C21   VSS_MAIN   NC
C23   VSS_MAIN   NC
C25   VSS_MAIN   VDD_PCIE1_1P0
C27   VSS_MAIN   VDD_PCIE0_1P0
C29   VSS_MAIN   NC
C31   VSS_MAIN   NC
C33   VSS_MAIN   NC
C35   VSS_MAIN   VDD_ANA0_1P8
C37   VSS_MAIN   VDDUSBOTG2_3P3
C39   VSS_MAIN   VDDUSBOTG1_3P3
C41   VSS_MAIN   NC
C43   VSS_MAIN   NC
C45   VSS_MAIN   VDD_ENET0
C47   VSS_MAIN   VDD_ENET1
C49   VSS_MAIN   NC
C51   VSS_MAIN   VDD_ENET1
C53   VSS_MAIN   NC
D2   VSS_MAIN   VDDMLBDIG
D6   VSS_MAIN   NC
D8   VSS_MAIN   VDDUSDHCVSELECT
D10   VSS_MAIN   VDDENET_MDIO
D12   VSS_MAIN   VDDQSPI1A
D14   VSS_MAIN   VDDQSPI1A
D16   VSS_MAIN   NC
D18   VSS_MAIN   NC
D20   VSS_MAIN   VDDPCIE_DIG
D22   NC   NC
D24   VSS_MAIN   NC
D26   VSS_MAIN   NC
D28   VSS_MAIN   NC
D30   VSS_MAIN   VDD_MLB_1P8
D32   VSS_MAIN   VDD_MLB_1P8
D34   VSS_MAIN   NC
D36   VSS_MAIN   NC
D38   VSS_MAIN   NC
D40   VSS_MAIN   NC
D42   VSS_MAIN   VDD_ENET0
D44   VSS_MAIN   VDD_ENET0
D46   VSS_MAIN   VDD_ENET1
D48   VSS_MAIN   VDD_ENET1
D52   VSS_MAIN   VDD_ENET1
E1   VSS_MAIN   VDDMLBDIG
E3   VSS_MAIN   VDDMLBDIG
E5   VSS_MAIN   VDDFLEXCAN
E7   VSS_MAIN   VDDFLEXCAN
E9   VSS_MAIN   NC
E11   VSS_MAIN   VDDQSPI1A
E13   VSS_MAIN   VDDQSPI1A
E15   VSS_MAIN   VDDQSPI0
E17   VSS_MAIN   VDDQSPI0
E19   VSS_MAIN   NC
E21   VSS_MAIN   NC
E23   NC   NC
E25   NC   NC
E27   NC   NC
E29   NC   NC
E31   VSS_MAIN   VDD_MLB_1P8
E33   VSS_MAIN   VDD_MLB_1P8
E35   VSS_MAIN   VDD_MLB_1P8
E37   VSS_MAIN   VDDUSDHC1
E39   VSS_MAIN   VDDUSDHC1
E41   VSS_MAIN   VDD_ENET0
E43   VSS_MAIN   VDD_ENET0
E45   VSS_MAIN   VDD_ENET0
E47   VSS_MAIN   NC
E49   VSS_MAIN   VDD_ENET1
E51   VSS_MAIN   VDD_ENET1
E53   VSS_MAIN   VDD_ENET1
F2   VSS_MAIN   NC
F4   VSS_MAIN   NC
F8   VSS_MAIN   VDDUSBSS3TC
F10   VSS_MAIN   VDDQSPI1A
F12   VSS_MAIN   NC
F14   VSS_MAIN   VDDQSPI0
F16   VSS_MAIN   VDDQSPI0
F18   VSS_MAIN   VDDQSPI0
F20   VSS_MAIN   VDDQSPI0
F22   VSS_MAIN   VDDQSPI0
F24   VSS_MAIN   NC
F26   NC   NC
F28   VSS_MAIN   VDD_USB_HSIC0
F30   NC   NC
F32   VSS_MAIN   NC
F34   VSS_MAIN   VDD_MLB_1P8
F36   VSS_MAIN   NC
F38   VSS_MAIN   VDDUSDHC1
F40   VSS_MAIN   VDDUSDHC1
F42   VSS_MAIN   VDDUSDHC1
F44   VSS_MAIN   NC
F46   VSS_MAIN   VDD_USDHC2
F50   VSS_MAIN   NC
F52   VSS_MAIN   NC
G1   VSS_MAIN   VDDRCH1_VDDQ
G3   VSS_MAIN   VDDRCH1_VDDQ
G5   VSS_MAIN   NC
G7   VSS_MAIN   VDDFLEXCAN
G9   VSS_MAIN   NC
G11   VSS_MAIN   VDDQSPI1A
G13   VSS_MAIN   VDDQSPI0
G15   VSS_MAIN   NC
G17   VSS_MAIN   VDDQSPI0
G19   VSS_MAIN   VDDQSPI0
G21   VSS_MAIN   NC
G23   VSS_MAIN   NC
G25   VSS_MAIN   VDDPCIE_DIG
G27   VSS_MAIN   NC
G29   VSS_MAIN   VDD_EMMC0
G31   VSS_MAIN   VDD_EMMC0
G33   VSS_MAIN   NC
G35   VSS_MAIN   VDD_EMMC0
G37   VSS_MAIN   VDD_EMMC0
G39   VSS_MAIN   NC
G41   VSS_MAIN   VDDUSDHC1
G43   VSS_MAIN   VDDUSDHC1
G45   VSS_MAIN   VDD_USDHC2
G47   VSS_MAIN   VDD_ENET1
G49   VSS_MAIN   NC
G51   VSS_MAIN   VDDRCH0_VDDQ
G53   VSS_MAIN   VDDRCH0_VDDQ
H2   VSS_MAIN   VDDRCH1_VDDQ
H4   VSS_MAIN   VDDRCH1_VDDQ
H6   VSS_MAIN   VDDFLEXCAN
H10   VSS_MAIN   VDDUSBSS3TC
H12   VSS_MAIN   VDDQSPI1A
H14   VSS_MAIN   VDDQSPI0
H16   VSS_MAIN   VDDQSPI0
H18   VSS_MAIN   VDDQSPI0
H20   VSS_MAIN   VDDQSPI0
H22   VSS_MAIN   VDDQSPI0
H24   VSS_MAIN   VDDQSPI0
H26   VSS_MAIN   VDD_USB_HSIC0
H28   VSS_MAIN   VDD_EMMC0
H30   VSS_MAIN   VDD_EMMC0
H32   VSS_MAIN   VDD_EMMC0
H34   VSS_MAIN   VDD_EMMC0
H36   VSS_MAIN   VDD_EMMC0
H38   VSS_MAIN   VDD_EMMC0
H40   VSS_MAIN   VDDUSDHC1
H42   VSS_MAIN   VDDUSDHC1
H44   VSS_MAIN   VDD_USDHC2
H48   VSS_MAIN   VDD_USDHC2
H50   VSS_MAIN   VDDRCH0_VDDQ
H52   VSS_MAIN   VDDRCH0_VDDQ
J1   VSS_MAIN   NC
J3   VSS_MAIN   NC
J5   VSS_MAIN   NC
J7   VSS_MAIN   NC
J9   VSS_MAIN   VDDUSBSS3TC
J11   VSS_MAIN   VDDQSPI1A
J13   VSS_MAIN   NC
J15   VSS_MAIN   NC
J17   VSS_MAIN   NC
J19   VSS_MAIN   NC
J21   VSS_MAIN   NC
J23   VSS_MAIN   NC
J25   VSS_MAIN   NC
J27   VSS_MAIN   VDD_EMMC0
J29   VSS_MAIN   NC
J31   VSS_MAIN   NC
J33   VSS_MAIN   VDD_EMMC0
J35   VSS_MAIN   NC
J37   VSS_MAIN   NC
J39   VSS_MAIN   VDDUSDHC1
J41   VSS_MAIN   NC
J43   VSS_MAIN   VDDUSDHC1
J45   VSS_MAIN   VDD_USDHC2
J47   VSS_MAIN   NC
J49   VSS_MAIN   NC
J51   VSS_MAIN   NC
J53   VSS_MAIN   NC
K2   VSS_MAIN   VDDRCH1_VDDQ
K4   VSS_MAIN   VDDRCH1_VDDQ
K6   VSS_MAIN   VDDRCH1_VDDQ
K8   VSS_MAIN   NC
K12   VSS_MAIN   NC
K14   VSS_MAIN   NC
K16   VSS_MAIN   NC
K18   VSS_MAIN   NC
K20   VSS_MAIN   NC
K22   VSS_MAIN   NC
K24   VSS_MAIN   NC
K26   VSS_MAIN   NC
K28   VSS_MAIN   NC
K30   VSS_MAIN   NC
K32   VSS_MAIN   NC
K34   VSS_MAIN   NC
K36   VSS_MAIN   NC
K38   VSS_MAIN   NC
K40   VSS_MAIN   NC
K42   VSS_MAIN   NC
K46   VSS_MAIN   NC
K48   VSS_MAIN   VDDRCH0_VDDQ
K50   VSS_MAIN   VDDRCH0_VDDQ
K52   VSS_MAIN   VDDRCH0_VDDQ
L1   VSS_MAIN   VDDRCH1_VDDQ
L3   VSS_MAIN   VDDRCH1_VDDQ
L5   VSS_MAIN   VDDRCH1_VDDQ
L7   VSS_MAIN   VDDRCH1_VDDQ
L9   VSS_MAIN   VDDUSBSS3TC
L11   VSS_MAIN   NC
L13   VSS_MAIN   NC
L15   VSS_MAIN   NC
L17   VSS_MAIN   NC
L19   VSS_MAIN   NC
L21   VSS_MAIN   NC
L23   VSS_MAIN   NC
L25   VSS_MAIN   NC
L27   VSS_MAIN   NC
L29   VSS_MAIN   NC
L31   VSS_MAIN   NC
L33   VSS_MAIN   NC
L35   VSS_MAIN   NC
L37   VSS_MAIN   NC
L39   VSS_MAIN   NC
L41   VSS_MAIN   NC
L43   VSS_MAIN   NC
L45   VSS_MAIN   VDD_USDHC2
L47   VSS_MAIN   VDDRCH0_VDDQ
L49   VSS_MAIN   VDDRCH0_VDDQ
L51   VSS_MAIN   VDDRCH0_VDDQ
L53   VSS_MAIN   VDDRCH0_VDDQ
M2   VSS_MAIN   NC
M4   VSS_MAIN   NC
M6   VSS_MAIN   NC
M8   VSS_MAIN   NC
M10   VSS_MAIN   NC
M14   NC   VDDMLBDIG
M16   NC   VDDUSBSS3TC
M18   NC   VDDQSPI1A
M20   SATA0PLLREFRET  NC
M22   NC   VDDPCIE1PLL_1P8
M24   NC   VDD_SATA0_1P0
M26   NC   VDD_PCIE0_1P0
M28   PCIE0PLLREFRET  NC
M30   NC   VDUSBSS3LDO_CAP
M32   NC   VDDUSBOTG1_1P0
M34   NC   VDDUSBOTG2_3P3
M36   NC   VDDUSDHC1
M38   NC   VDD_USDHC2
M40   NC   VDD_ENET0
M44   VSS_MAIN   NC
M46   VSS_MAIN   NC
M48   VSS_MAIN   NC
M50   VSS_MAIN   NC
M52   VSS_MAIN   NC
N1   VSS_MAIN   VDDRCH1_VDDQ
N3   VSS_MAIN   VDDRCH1_VDDQ
N5   VSS_MAIN   VDDRCH1_VDDQ
N7   VSS_MAIN   VDDRCH1_VDDQ
N9   VSS_MAIN   VDDRCH1_VDDQ
N11   VSS_MAIN   VDDRCH1_VDDQ
N13   VSS_MAIN   NC
N15   NC   VDDFLEXCAN
N17   NC   VDDENET_MDIO
N19   NC   VDDQSPI0
N21   NC   VDDSATA0PLL_1P8
N23   PCIE1PLLREFRET  NC
N25   NC   VDD_PCIE1_1P0
N27   NC   VDDPCIE0PLL_1P8
N29   NC   VDDPCIELDO_CAP
N31   NC   VDDUSBOTG2_1P0
N33   NC   VDDUSBOTG1_3P3
N35   NC   VDD_EMMC0
N37   NC   VDDUSDHC1
N39   NC   VDD_ENET0
N41   VSS_MAIN   NC
N43   VSS_MAIN   VDDRCH0_VDDQ
N45   VSS_MAIN   VDDRCH0_VDDQ
N47   VSS_MAIN   VDDRCH0_VDDQ
N49   VSS_MAIN   VDDRCH0_VDDQ
N51   VSS_MAIN   VDDRCH0_VDDQ
N53   VSS_MAIN   VDDRCH0_VDDQ
P2   VSS_MAIN   VDDRCH1_VDDQ
P4   VSS_MAIN   VDDRCH1_VDDQ
P6   VSS_MAIN   VDDRCH1_VDDQ
P8   VSS_MAIN   VDDRCH1_VDDQ
P10   VSS_MAIN   VDDRCH1_VDDQ
P12   VSS_MAIN   NC
P42   VSS_MAIN   NC
P44   VSS_MAIN   VDDRCH0_VDDQ
P46   VSS_MAIN   VDDRCH0_VDDQ
P48   VSS_MAIN   VDDRCH0_VDDQ
P50   VSS_MAIN   VDDRCH0_VDDQ
P52   VSS_MAIN   VDDRCH0_VDDQ
R1   VSS_MAIN   NC
R3   VSS_MAIN   NC
R5   VSS_MAIN   NC
R7   VSS_MAIN   NC
R9   VSS_MAIN   NC
R11   VSS_MAIN   NC
R15   VSS_MAIN   NC
R17   VSS_MAIN   NC
R19   VSS_MAIN   NC
R21   VSS_MAIN   NC
R23   VSS_MAIN   NC
R25   VSS_MAIN   NC
R27   VSS_MAIN   NC
R29   VSS_MAIN   NC
R31   VSS_MAIN   NC
R33   VSS_MAIN   NC
R35   VSS_MAIN   NC
R37   VSS_MAIN   NC
R39   VSS_MAIN   NC
R43   VSS_MAIN   NC
R45   VSS_MAIN   NC
R47   VSS_MAIN   NC
R49   VSS_MAIN   NC
R51   VSS_MAIN   NC
R53   VSS_MAIN   NC
T2   VSS_MAIN   VDDRCH1_VDDQ
T4   VSS_MAIN   VDDRCH1_VDDQ
T6   VSS_MAIN   VDDRCH1_VDDQ
T8   VSS_MAIN   VDDRCH1_VDDQ
T10   VSS_MAIN   VDDRCH1_VDDQ
T12   VSS_MAIN   NC
T16   VSS_MAIN   NC
T18   NC   VDDUSDHCVSELECT
T20   VSS_MAIN   NC
T22   NC   VDDPCIE_DIG
T24   VSS_MAIN   NC
T26   NC   VDDPCIEIOB_1P8
T28   VSS_MAIN   NC
T30   NC   VDD_MLB_1P8
T32   VSS_MAIN   NC
T34   NC   VDD_MAIN
T36   VSS_MAIN   NC
T38   NC   VDD_ENET1
T42   VSS_MAIN   NC
T44   VSS_MAIN   VDDRCH0_VDDQ
T46   VSS_MAIN   VDDRCH0_VDDQ
T48   VSS_MAIN   VDDRCH0_VDDQ
T50   VSS_MAIN   VDDRCH0_VDDQ
T52   VSS_MAIN   VDDRCH0_VDDQ
U1   VSS_MAIN   VDDRCH1_VDDQCKE
U3   VSS_MAIN   VDDRCH1_VDDQ
U5   VSS_MAIN   VDDRCH1_VDDQ
U7   VSS_MAIN   VDDRCH1_VDDQCKE
U9   VSS_MAIN   VDDRCH1_VDDQ
U11   NC   NC
U15   NC   VDDRCH1_VDDQ
U17   VSS_MAIN   NC
U19   NC   VDD_MAIN
U21   VSS_MAIN   NC
U23   NC   VDD_MAIN
U25   NC   VDD_ANA1_1P8
U27   NC   VDDPCIELDO_1P8
U29   NC   VDD_ANA0_1P8
U31   NC   VDD_ANA0_1P8
U33   VSS_MAIN   NC
U35   NC   VDD_GPU1
U37   VSS_MAIN   NC
U39   NC   VDDRCH0_VDDQ
U43   NC   NC
U45   VSS_MAIN   VDDRCH0_VDDQ
U47   VSS_MAIN   VDDRCH0_VDDQCKE
U49   VSS_MAIN   VDDRCH0_VDDQ
U51   VSS_MAIN   VDDRCH0_VDDQ
U53   VSS_MAIN   VDDRCH0_VDDQCKE
V2   VSS_MAIN   NC
V4   VSS_MAIN   NC
V6   VSS_MAIN   NC
V8   VSS_MAIN   NC
V10   VSS_MAIN   NC
V12   VSS_MAIN   NC
V16   NC   VDDRCH1_VDDQ
V18   VSS_MAIN   NC
V20   NC   VDD_GPU0
V22   VSS_MAIN   NC
V24   NC   VDD_MAIN
V26   NC   VDD_USB_HSIC0
V28   NC   VDD_USB_HSIC0
V30   VSS_MAIN   NC
V32   NC   VDD_MAIN
V34   VSS_MAIN   NC
V36   NC   VDD_GPU1
V38   NC   VDDRCH0_VDDQ
V42   VSS_MAIN   NC
V44   VSS_MAIN   NC
V46   VSS_MAIN   NC
V48   VSS_MAIN   NC
V50   VSS_MAIN   NC
V52   VSS_MAIN   NC
W1   VSS_MAIN   VDDRCH1_VDDQCKE
W3   VSS_MAIN   VDDRCH1_VDDQCKE
W5   VSS_MAIN   VDDRCH1_VDDQCKE
W7   VSS_MAIN   VDDRCH1_VDDQCKE
W9   VSS_MAIN   VDDRCH1_VDDQCKE
W11   VSS_MAIN   VDDRCH1_VDDQCKE
W15   NC   VDDRCH1_VDDQ
W17   NC   VDD_MEMC
W19   VSS_MAIN   NC
W21   NC   VDD_GPU0
W23   VSS_MAIN   NC
W25   NC   VDD_MAIN
W27   VSS_MAIN   NC
W29   NC   VDD_MAIN
W31   VSS_MAIN   NC
W33   NC   VDD_GPU1
W35   VSS_MAIN   NC
W37   NC   VDD_MEMC
W39   NC   VDDRCH0_VDDQ
W43   VSS_MAIN   VDDRCH0_VDDQCKE
W45   VSS_MAIN   VDDRCH0_VDDQCKE
W47   VSS_MAIN   VDDRCH0_VDDQCKE
W49   VSS_MAIN   VDDRCH0_VDDQCKE
W51   VSS_MAIN   VDDRCH0_VDDQCKE
W53   VSS_MAIN   VDDRCH0_VDDQCKE
Y2   VSS_MAIN   VDDRCH1_VDDQCKE
Y4   VSS_MAIN   VDDRCH1_VDDQCKE
Y6   VSS_MAIN   VDDRCH1_VDDQCKE
Y8   VSS_MAIN   VDDRCH1_VDDQCKE
Y10   VSS_MAIN   VDDRCH1_VDDQCKE
Y12   VSS_MAIN   NC
Y16   NC   VDDRCH1_VDDQ
Y18   NC   VDD_GPU0
Y20   VSS_MAIN   NC
Y22   NC   VDD_GPU0
Y24   VSS_MAIN   NC
Y26   NC   VDD_MAIN
Y28   VSS_MAIN   NC
Y30   NC   VDD_MAIN
Y32   VSS_MAIN   NC
Y34   NC   VDD_GPU1
Y36   VSS_MAIN   NC
Y38   NC   VDDRCH0_VDDQ
Y42   VSS_MAIN   NC
Y44   VSS_MAIN   VDDRCH0_VDDQCKE
Y46   VSS_MAIN   VDDRCH0_VDDQCKE
Y48   VSS_MAIN   VDDRCH0_VDDQCKE
Y50   VSS_MAIN   VDDRCH0_VDDQCKE
Y52   VSS_MAIN   VDDRCH0_VDDQCKE
AA1   VSS_MAIN   NC
AA3   VSS_MAIN   NC
AA5   VSS_MAIN   NC
AA7   VSS_MAIN   NC
AA9   VSS_MAIN   NC
AA11   VSS_MAIN   NC
AA13   VSS_MAIN   NC
AA15   NC   VDDRCH1_VDDQ
AA17   VSS_MAIN   NC
AA19   NC   VDD_GPU0
AA21   VSS_MAIN   NC
AA23   NC   VDD_MAIN
AA25   VSS_MAIN   NC
AA27   NC   VDD_MAIN
AA29   VSS_MAIN   NC
AA31   NC   VDD_MAIN
AA33   VSS_MAIN   NC
AA35   NC   VDD_GPU1
AA37   VSS_MAIN   NC
AA39   NC   VDDRCH0_VDDQ
AA41   VSS_MAIN   NC
AA43   VSS_MAIN   NC
AA45   VSS_MAIN   NC
AA47   VSS_MAIN   NC
AA49   VSS_MAIN   NC
AA51   VSS_MAIN   NC
AA53   VSS_MAIN   NC
AB2   VSS_MAIN   VDDRCH1_VDDQCKE
AB4   VSS_MAIN   VDDRCH1_VDDQCKE
AB6   VSS_MAIN   VDDRCH1_VDDQCKE
AB8   VSS_MAIN   VDDRCH1_VDDQCKE
AB10   VSS_MAIN   VDDRCH1_VDDQCKE
AB12   VSS_MAIN   NC
AB16   NC   VDDRCH1_VDDQCKE
AB18   VSS_MAIN   NC
AB20   NC   VDD_GPU0
AB22   VSS_MAIN   NC
AB24   NC   VDD_MAIN
AB26   VSS_MAIN   NC
AB28   NC   VDD_MAIN
AB30   VSS_MAIN   NC
AB32   NC   VDD_GPU1
AB34   VSS_MAIN   NC
AB36   NC   VDD_GPU1
AB38   NC   VDDRCH0_VDDQCKE
AB42   VSS_MAIN   NC
AB44   VSS_MAIN   VDDRCH0_VDDQCKE
AB46   VSS_MAIN   VDDRCH0_VDDQCKE
AB48   VSS_MAIN   VDDRCH0_VDDQCKE
AB50   VSS_MAIN   VDDRCH0_VDDQCKE
AB52   VSS_MAIN   VDDRCH0_VDDQCKE
AC1   VSS_MAIN   VDDRCH1_VDDQCKE
AC3   VSS_MAIN   VDDRCH1_VDDQCKE
AC5   VSS_MAIN   VDDRCH1_VDDQCKE
AC7   VSS_MAIN   VDDRCH1_VDDQCKE
AC9   VSS_MAIN   VDDRCH1_VDDQCKE
AC11   VSS_MAIN   VDDRCH1_VDDQCKE
AC13   VSS_MAIN   NC
AC15   NC   VDDRCH1_VDDQCKE
AC17   NC   VDD_MEMC
AC19   VSS_MAIN   NC
AC21   NC   VDD_GPU0
AC23   VSS_MAIN   NC
AC25   NC   VDD_MAIN
AC27   VSS_MAIN   NC
AC29   NC   VDD_MAIN
AC31   VSS_MAIN   NC
AC33   NC   VDD_GPU1
AC35   VSS_MAIN   NC
AC37   NC   VDD_MEMC
AC39   NC   VDDRCH0_VDDQCKE
AC41   VSS_MAIN   NC
AC43   VSS_MAIN   VDDRCH0_VDDQCKE
AC45   VSS_MAIN   VDDRCH0_VDDQCKE
AC47   VSS_MAIN   VDDRCH0_VDDQCKE
AC49   VSS_MAIN   VDDRCH0_VDDQCKE
AC51   VSS_MAIN   VDDRCH0_VDDQCKE
AC53   VSS_MAIN   VDDRCH0_VDDQCKE
AD2   VSS_MAIN   NC
AD4   VSS_MAIN   NC
AD6   VSS_MAIN   NC
AD8   VSS_MAIN   NC
AD10   VSS_MAIN   NC
AD12   VSS_MAIN   NC
AD16   NC   VDDRCH1_VDDQCKE
AD18   NC   VDD_GPU0
AD20   VSS_MAIN   NC
AD22   NC   VDD_GPU0
AD24   VSS_MAIN   NC
AD26   NC   VDD_MAIN
AD28   VSS_MAIN   NC
AD30   NC   VDD_MAIN
AD32   VSS_MAIN   NC
AD34   NC   VDD_GPU1
AD36   VSS_MAIN   NC
AD38   NC   VDDRCH0_VDDQCKE
AD42   VSS_MAIN   NC
AD44   VSS_MAIN   NC
AD46   VSS_MAIN   NC
AD48   VSS_MAIN   NC
AD50   VSS_MAIN   NC
AD52   VSS_MAIN   NC
AE1   VSS_MAIN   VDDRCH1_VDDQCKE
AE3   VSS_MAIN   VDDRCH1_VDDQ
AE5   VSS_MAIN   VDDRCH1_VDDQ
AE7   VSS_MAIN   VDDRCH1_VDDQ
AE9   VSS_MAIN   VDDRCH1_VDDQCKE
AE11   NC   VDDRCH1_VDDAPLL
AE13   VSS_MAIN   NC
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[Diff Pin]  inv_pin  vdiff  tdelay_typ tdelay_min tdelay_max
A19   B20   NA   NA   NA   NA
A21   B22   NA   NA   NA   NA
A29   B30   NA   NA   NA   NA
A33   B32   NA   NA   NA   NA
B16   C17   NA   NA   NA   NA
B24   C25   NA   NA   NA   NA
B26   C27   NA   NA   NA   NA
B38   C37   NA   NA   NA   NA
B40   C39   NA   NA   NA   NA
C35   B34   NA   NA   NA   NA
D30   E31   NA   NA   NA   NA
D32   E33   NA   NA   NA   NA
F34   E35   NA   NA   NA   NA
K2   L1   NA   NA   NA   NA
K52   L53   NA   NA   NA   NA
N1   P2   NA   NA   NA   NA
N53   P52   NA   NA   NA   NA
W5   Y4   NA   NA   NA   NA
W49   Y50   NA   NA   NA   NA
AC5   AB4   NA   NA   NA   NA
AC49   AB50   NA   NA   NA   NA
AJ1   AH2   NA   NA   NA   NA
AJ53   AH52   NA   NA   NA   NA
AM2   AL1   NA   NA   NA   NA
AM52   AL53   NA   NA   NA   NA
BF16   BE17   NA   NA   NA   NA
BF18   BE19   NA   NA   NA   NA
BF20   BE21   NA   NA   NA   NA
BF22   BE23   NA   NA   NA   NA
BF24   BE25   NA   NA   NA   NA
BG27   BH26   NA   NA   NA   NA
BG29   BH28   NA   NA   NA   NA
BG31   BH30   NA   NA   NA   NA
BG33   BH32   NA   NA   NA   NA
BG35   BH34   NA   NA   NA   NA
BH2   BG3   NA   NA   NA   NA
BH38   BG37   NA   NA   NA   NA
BH40   BG39   NA   NA   NA   NA
BH42   BG41   NA   NA   NA   NA
BH44   BG43   NA   NA   NA   NA
BH46   BG45   NA   NA   NA   NA
BJ13   BH12   NA   NA   NA   NA
BJ15   BH14   NA   NA   NA   NA
BJ17   BH16   NA   NA   NA   NA
BJ19   BH18   NA   NA   NA   NA
BJ21   BH20   NA   NA   NA   NA
BK26   BM26   NA   NA   NA   NA
BK28   BM28   NA   NA   NA   NA
BL3   BK2   NA   NA   NA   NA
BL5   BM4   NA   NA   NA   NA
BL7   BM6   NA   NA   NA   NA
BL9   BM8   NA   NA   NA   NA
BL25   BN25   NA   NA   NA   NA
BL27   BN27   NA   NA   NA   NA
BL29   BN29   NA   NA   NA   NA
BM12   BL11   NA   NA   NA   NA
BM14   BL13   NA   NA   NA   NA
BM16   BL15   NA   NA   NA   NA
BM18   BL17   NA   NA   NA   NA
BM20   BL19   NA   NA   NA   NA
BM30   BK30   NA   NA   NA   NA
BM32   BK32   NA   NA   NA   NA
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| Models and submodels in the file (264): BDPROGSCARUDQP_SDMMC_3V3SF_00_MMC (I/O), BDPROGSCARUDQP_SDMMC_3V3SF_00_SD (I/O), BDPROGSCARUDQP_SDMMC_3V3SF_01_MMC (I/O), BDPROGSCARUDQP_SDMMC_3V3SF_01_SD (I/O), BDPROGSCARUDQP_SDMMC_3V3SF_10 (I/O), BDPROGSCARUDQP_SDMMC_3V3SF_10_2v7 (I/O), BDPROGSCARUDQP_SDMMC_3V3SF_11 (I/O), BDPROGSCARUDQP_SDMMC_3V3SF_11_2v7 (I/O), BDPROG_00 (I/O), BDPROG_01 (I/O), BDPROG_10 (I/O), BDPROG_11 (I/O), BD_10mA (I/O), BD_12mA (I/O), BD_1mA (I/O), BD_2mA (I/O), BD_4mA (I/O), BD_6mA (I/O), BD_8mA (I/O), BD_HS (I/O), DWC_D5MC3L_34 (I/O), DWC_D5MC3L_40 (I/O), DWC_D5MC3L_48 (I/O), DWC_D5MC3L_ODT40 (Input), DWC_D5MC3L_ODT60 (Input), DWC_D5MC3L_ODTOFF (Input), DWC_D5MC3_34 (I/O), DWC_D5MC3_40 (I/O), DWC_D5MC3_48 (I/O), DWC_D5MC3_ODT40 (Input), DWC_D5MC3_ODT60 (Input), DWC_D5MC3_ODTOFF (Input), DWC_D5MC4_34 (I/O), DWC_D5MC4_34M (I/O), DWC_D5MC4_34M_TXM (I/O), DWC_D5MC4_34ODT40 (Input), DWC_D5MC4_34ODTOFF (Input), DWC_D5MC4_34_TXM (I/O), DWC_D5MC4_48 (I/O), DWC_D5MC4_48M (I/O), DWC_D5MC4_48M_TXM (I/O), DWC_D5MC4_48ODT60 (Input), DWC_D5MC4_48_TXM (I/O), DWC_D5MCK3L_34 (I/O), DWC_D5MCK3L_40 (I/O), DWC_D5MCK3L_48 (I/O), DWC_D5MCK3L_ODT40 (Input), DWC_D5MCK3L_ODT60 (Input), DWC_D5MCK3L_ODTOFF (Input), DWC_D5MCK3_34 (I/O), DWC_D5MCK3_40 (I/O), DWC_D5MCK3_48 (I/O), DWC_D5MCK3_ODT40 (Input), DWC_D5MCK3_ODT60 (Input), DWC_D5MCK3_ODTOFF (Input), DWC_D5MCK4_34 (I/O), DWC_D5MCK4_34M (I/O), DWC_D5MCK4_34M_TXM (I/O), DWC_D5MCK4_34ODT40 (Input), DWC_D5MCK4_34ODTOFF (Input), DWC_D5MCK4_34_TXM (I/O), DWC_D5MCK4_48 (I/O), DWC_D5MCK4_48M (I/O), DWC_D5MCK4_48M_TXM (I/O), DWC_D5MCK4_48ODT60 (Input), DWC_D5MCK4_48_TXM (I/O), DWC_D5MCKL2_34 (I/O), DWC_D5MCKL2_48 (I/O), DWC_D5MCKL2_ODTOFF (Input), DWC_D5MCKL3_34 (I/O), DWC_D5MCKL3_34M (I/O), DWC_D5MCKL3_34ODT120 (Input), DWC_D5MCKL3_34ODT240 (Input), DWC_D5MCKL3_34ODT60 (Input), DWC_D5MCKL3_34ODTOFF (Input), DWC_D5MCKL3_40 (I/O), DWC_D5MCKL3_48 (I/O), DWC_D5MCKL3_48M (I/O), DWC_D5MCKL3_ODT120M (Input), DWC_D5MCKL3_ODT240M (Input)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
